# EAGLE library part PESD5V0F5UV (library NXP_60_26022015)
Femtofarad unidirectional fivefold ESD protection array Femtofarad capacitance unidirectional ElectroStatic Discharge (ESD) protection diode array designed to protect up to five signal lines from the damage caused by ESD and other transients. The device is encapsulated in an ultra small and flat lead SOT666 Surface-Mounted Device (SMD) plastic package. The combination of extremely low capacitance, high ESD maximum rating and ultra small package makes the device ideal for high-speed data line protection and antenna protection applications. AAL Eindhoven MK
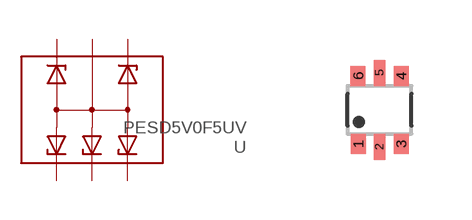
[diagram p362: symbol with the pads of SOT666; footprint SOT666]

Designator prefix U

## PESD5V0F5UV  [SOT666]
1  K1  pas
2  CA  pas
3  K2  pas
4  K3  pas
5  K4  pas
6  K5  pas

## Footprint SOT666 (pad centres in mm)
SOT 666 Reflow soldering foorprint Source: Philips - BAS70_1PS7XSB70_SER_8.pdf
smd 0.375 x 0.5: 1 -0.537,-0.85; 3 0.538,-0.85; 4 0.538,0.85; 6 -0.538,0.85
smd 0.3 x 0.65: 2 0,-0.925; 5 0,0.925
